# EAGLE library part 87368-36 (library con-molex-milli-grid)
RECEPTACAL
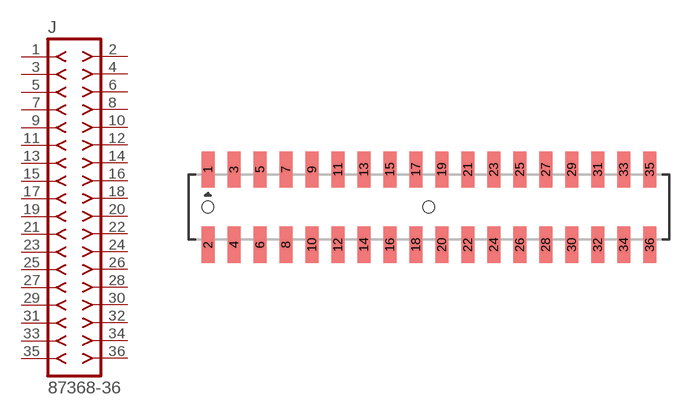
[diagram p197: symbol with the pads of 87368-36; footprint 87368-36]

Designator prefix J

## 87368-36  [87368-36]
1  1  pas
2  2  pas
3  3  pas
4  4  pas
5  5  pas
6  6  pas
7  7  pas
8  8  pas
9  9  pas
10  10  pas
11  11  pas
12  12  pas
13  13  pas
14  14  pas
15  15  pas
16  16  pas
17  17  pas
18  18  pas
19  19  pas
20  20  pas
21  21  pas
22  22  pas
23  23  pas
24  24  pas
25  25  pas
26  26  pas
27  27  pas
28  28  pas
29  29  pas
30  30  pas
31  31  pas
32  32  pas
33  33  pas
34  34  pas
35  35  pas
36  36  pas

## Footprint 87368-36 (pad centres in mm)
RECEPTACAL SMD Dual Row, Side Entry
smd 1 x 2.8: 1 -17,2.9; 2 -17,-2.9; 3 -15,2.9; 4 -15,-2.9; 5 -13,2.9; 6 -13,-2.9; 7 -11,2.9; 8 -11,-2.9; 9 -9,2.9; 10 -9,-2.9; 11 -7,2.9; 12 -7,-2.9; 13 -5,2.9; 14 -5,-2.9; 15 -3,2.9; 16 -3,-2.9; 17 -1,2.9; 18 -1,-2.9; 19 1,2.9; 20 1,-2.9; 21 3,2.9; 22 3,-2.9; 23 5,2.9; 24 5,-2.9; 25 7,2.9; 26 7,-2.9; 27 9,2.9; 28 9,-2.9; 29 11,2.9; 30 11,-2.9; 31 13,2.9; 32 13,-2.9; 33 15,2.9; 34 15,-2.9; 35 17,2.9; 36 17,-2.9
hole 0.914 at -17,0
hole 0.914 at 0,0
